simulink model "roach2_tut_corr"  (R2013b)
settings: Solver=VariableStepDiscrete  SolverMode=SingleTasking  StartTime=0.0  StopTime=100  RelTol=1e-3
undefined symbols (not defined in the file): add_latency, addr_width, Bit, bitfield, BitWidth, bram_latency, burst_size, casper_library_scopes, conv_latency, data_width, DelayLen, fan_latency, FFTSize, FFTStage, getfield, increment, led, Location, Lower, mult_latency, mux_latency, n_bits, n_bits_data, n_inputs, n_streams, n_taps, neg_latency, negate_latency, nsamples, pfb_size, pulse_len, reset_period, ROACH, ROACH2, snapshot, sx475t, sync_period, sync_period_bits, Upper, UseCounter, Width
libraries: xbsIndex_r4 x24444, casper_library_misc x73, xbsReplacements_r4 x34, casper_library_delays x14, xps_library x7
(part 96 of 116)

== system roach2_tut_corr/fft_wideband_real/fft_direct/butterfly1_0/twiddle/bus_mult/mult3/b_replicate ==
  in : Inport
  bussify : Subsystem  AncestorBlock=casper_library_flow_control/bus_create
  din0_0 : xbsIndex_r4/Delay  rst=off  infoeditControl=Selection of Reset will increase slice count due to use of real FFs and instead of SRLs  en=off  latency=1  dbl_ovrd=off  reg_retiming=off  block_type=delay
  din0_1 : xbsIndex_r4/Delay  rst=off  infoeditControl=Selection of Reset will increase slice count due to use of real FFs and instead of SRLs  en=off  latency=1  dbl_ovrd=off  reg_retiming=off  block_type=delay
  out : Outport
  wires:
  in/1 -> din0_0/1, din0_1/1
  din0_0/1 -> bussify/1(in1)
  din0_1/1 -> bussify/2(in2)
  bussify/1(bus_out) -> out/1

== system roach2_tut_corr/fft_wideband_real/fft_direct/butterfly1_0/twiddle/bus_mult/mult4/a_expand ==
  bus_in : Inport
  reinterpret{1..4} (4 alike) : xbsIndex_r4/Reinterpret  force_arith_type=on  arith_type="Signed  (2's comp)"  force_bin_pt=on  bin_pt=17  block_type=reinterpret
  slice1 : xbsIndex_r4/Slice  nbits=18  boolean_output=off  mode=Upper Bit Location + Width  bit1=-54  base1=MSB of Input  bit0=0  base0=LSB of Input  dbl_ovrd=off  block_type=slice
  slice2 : xbsIndex_r4/Slice  nbits=18  boolean_output=off  mode=Upper Bit Location + Width  bit1=-36  base1=MSB of Input  bit0=0  base0=LSB of Input  dbl_ovrd=off  block_type=slice
  slice3 : xbsIndex_r4/Slice  nbits=18  boolean_output=off  mode=Upper Bit Location + Width  bit1=-18  base1=MSB of Input  bit0=0  base0=LSB of Input  dbl_ovrd=off  block_type=slice
  slice4 : xbsIndex_r4/Slice  nbits=18  boolean_output=off  mode=Upper Bit Location + Width  bit1=0  base1=MSB of Input  bit0=0  base0=LSB of Input  dbl_ovrd=off  block_type=slice
  msb_out4 : Outport
  out3 : Outport  Port=2
  out2 : Outport  Port=3
  lsb_out1 : Outport  Port=4
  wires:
  bus_in/1 -> slice4/1, slice3/1, slice2/1, slice1/1
  slice4/1 -> reinterpret4/1
  reinterpret4/1 -> msb_out4/1
  slice3/1 -> reinterpret3/1
  reinterpret3/1 -> out3/1
  slice2/1 -> reinterpret2/1
  reinterpret2/1 -> out2/1
  slice1/1 -> reinterpret1/1
  reinterpret1/1 -> lsb_out1/1

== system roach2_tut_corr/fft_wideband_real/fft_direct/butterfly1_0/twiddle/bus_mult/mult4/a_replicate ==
  in : Inport
  bussify : Subsystem  AncestorBlock=casper_library_flow_control/bus_create
  din0_0 : xbsIndex_r4/Delay  rst=off  infoeditControl=Selection of Reset will increase slice count due to use of real FFs and instead of SRLs  en=off  latency=1  dbl_ovrd=off  reg_retiming=off  block_type=delay
  din0_1 : xbsIndex_r4/Delay  rst=off  infoeditControl=Selection of Reset will increase slice count due to use of real FFs and instead of SRLs  en=off  latency=1  dbl_ovrd=off  reg_retiming=off  block_type=delay
  out : Outport
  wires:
  in/1 -> din0_0/1, din0_1/1
  din0_0/1 -> bussify/1(in1)
  din0_1/1 -> bussify/2(in2)
  bussify/1(bus_out) -> out/1

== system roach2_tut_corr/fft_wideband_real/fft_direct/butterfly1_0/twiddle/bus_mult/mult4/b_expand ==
  bus_in : Inport
  reinterpret{1..4} (4 alike) : xbsIndex_r4/Reinterpret  force_arith_type=on  arith_type="Signed  (2's comp)"  force_bin_pt=on  bin_pt=17  block_type=reinterpret
  slice1 : xbsIndex_r4/Slice  nbits=18  boolean_output=off  mode=Upper Bit Location + Width  bit1=-54  base1=MSB of Input  bit0=0  base0=LSB of Input  dbl_ovrd=off  block_type=slice
  slice2 : xbsIndex_r4/Slice  nbits=18  boolean_output=off  mode=Upper Bit Location + Width  bit1=-36  base1=MSB of Input  bit0=0  base0=LSB of Input  dbl_ovrd=off  block_type=slice
  slice3 : xbsIndex_r4/Slice  nbits=18  boolean_output=off  mode=Upper Bit Location + Width  bit1=-18  base1=MSB of Input  bit0=0  base0=LSB of Input  dbl_ovrd=off  block_type=slice
  slice4 : xbsIndex_r4/Slice  nbits=18  boolean_output=off  mode=Upper Bit Location + Width  bit1=0  base1=MSB of Input  bit0=0  base0=LSB of Input  dbl_ovrd=off  block_type=slice
  msb_out4 : Outport
  out3 : Outport  Port=2
  out2 : Outport  Port=3
  lsb_out1 : Outport  Port=4
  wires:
  bus_in/1 -> slice4/1, slice3/1, slice2/1, slice1/1
  slice4/1 -> reinterpret4/1
  reinterpret4/1 -> msb_out4/1
  slice3/1 -> reinterpret3/1
  reinterpret3/1 -> out3/1
  slice2/1 -> reinterpret2/1
  reinterpret2/1 -> out2/1
  slice1/1 -> reinterpret1/1
  reinterpret1/1 -> lsb_out1/1

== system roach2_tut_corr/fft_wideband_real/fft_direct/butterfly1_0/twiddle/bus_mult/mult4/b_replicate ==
  in : Inport
  bussify : Subsystem  AncestorBlock=casper_library_flow_control/bus_create
  din0_0 : xbsIndex_r4/Delay  rst=off  infoeditControl=Selection of Reset will increase slice count due to use of real FFs and instead of SRLs  en=off  latency=1  dbl_ovrd=off  reg_retiming=off  block_type=delay
  din0_1 : xbsIndex_r4/Delay  rst=off  infoeditControl=Selection of Reset will increase slice count due to use of real FFs and instead of SRLs  en=off  latency=1  dbl_ovrd=off  reg_retiming=off  block_type=delay
  out : Outport
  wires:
  in/1 -> din0_0/1, din0_1/1
  din0_0/1 -> bussify/1(in1)
  din0_1/1 -> bussify/2(in2)
  bussify/1(bus_out) -> out/1

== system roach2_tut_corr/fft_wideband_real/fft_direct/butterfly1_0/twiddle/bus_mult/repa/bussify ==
  in1 : Inport
  reinterpret1 : xbsIndex_r4/Reinterpret  force_arith_type=on  arith_type=Unsigned  force_bin_pt=on  bin_pt=0  block_type=reinterpret
  bus_out : Outport
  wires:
  in1/1 -> reinterpret1/1
  reinterpret1/1 -> bus_out/1

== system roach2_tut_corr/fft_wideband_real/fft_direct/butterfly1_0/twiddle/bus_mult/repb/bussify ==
  in1 : Inport
  reinterpret1 : xbsIndex_r4/Reinterpret  force_arith_type=on  arith_type=Unsigned  force_bin_pt=on  bin_pt=0  block_type=reinterpret
  bus_out : Outport
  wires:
  in1/1 -> reinterpret1/1
  reinterpret1/1 -> bus_out/1

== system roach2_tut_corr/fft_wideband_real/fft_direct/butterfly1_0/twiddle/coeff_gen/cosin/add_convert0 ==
  theta : Inport
  misci : Inport  Port=2
  AddSub : xbsIndex_r4/AddSub  mode=Subtraction  use_carryin=off  use_carryout=off  en=off  latency=add_latency  precision=User Defined  arith_type=Unsigned  n_bits=10  bin_pt=0  quantization=Truncate  overflow=Wrap  dbl_ovrd=off  use_behavioral_HDL=off  hw_selection=Fabric  pipelined=on  block_type=addsub
  AddSub1 : xbsIndex_r4/AddSub  mode=Addition  use_carryin=off  use_carryout=off  en=off  latency=0  precision=User Defined  arith_type=Unsigned  n_bits=2  bin_pt=0  quantization=Truncate  overflow=Wrap  dbl_ovrd=off  use_behavioral_HDL=off  hw_selection=Fabric  pipelined=on  block_type=addsub
  AddSub5 : xbsIndex_r4/AddSub  mode=Addition  use_carryin=off  use_carryout=off  en=off  latency=0  precision=User Defined  arith_type=Unsigned  n_bits=2  bin_pt=0  quantization=Truncate  overflow=Wrap  dbl_ovrd=off  use_behavioral_HDL=off  hw_selection=Fabric  pipelined=off  block_type=addsub
  Concat : xbsIndex_r4/Concat  num_inputs=2  dbl_ovrd=off  block_type=concat
  Constant4 : xbsIndex_r4/Constant  const=512  gui_display_data_type=Fixed-point  arith_type=Unsigned  n_bits=10  bin_pt=0  preci_type=Single  exp_width=8  frac_width=24  explicit_period=off  period=1  equ=P=C  opselect=C  inp2=PCIN>>17  opr=+  inp1=P  carry=CIN  dbl_ovrd=off  block_type=constant
  Convert2 : xbsIndex_r4/Convert  gui_display_data_type=Fixed-point  arith_type=Unsigned  n_bits=9  bin_pt=0  float_type=Single  exp_bits=8  fraction_bits=24  quantization=Truncate  overflow=Saturate  en=off  latency=conv_latency  dbl_ovrd=off  pipeline=on  block_type=convert
  Delay1 : xbsIndex_r4/Delay  rst=off  infoeditControl=Selection of Reset will increase slice count due to use of real FFs and instead of SRLs  en=off  latency=mux_latency+add_latency+conv_latency  dbl_ovrd=off  reg_retiming=on  block_type=delay
  Delay13 : xbsIndex_r4/Delay  rst=off  infoeditControl=Selection of Reset will increase slice count due to use of real FFs and instead of SRLs  en=off  latency=add_latency  dbl_ovrd=off  reg_retiming=off  block_type=delay
  Delay14 : xbsIndex_r4/Delay  rst=off  infoeditControl=Selection of Reset will increase slice count due to use of real FFs and instead of SRLs  en=off  latency=add_latency  dbl_ovrd=off  reg_retiming=off  block_type=delay
  Delay2 : xbsIndex_r4/Delay  rst=off  infoeditControl=Selection of Reset will increase slice count due to use of real FFs and instead of SRLs  en=off  latency=add_latency+mux_latency+conv_latency  dbl_ovrd=off  reg_retiming=on  block_type=delay
  Mux : xbsIndex_r4/Mux  inputs=2  en=off  latency=mux_latency  precision=Full  arith_type=Unsigned  n_bits=16  bin_pt=14  quantization=Truncate  overflow=Wrap  dbl_ovrd=off  block_type=mux
  backwards : xbsIndex_r4/Slice  nbits=1  boolean_output=on  mode=Lower Bit Location + Width  bit1=0  base1=MSB of Input  bit0=0  base0=LSB of Input  dbl_ovrd=off  block_type=slice
  direction_offset : xbsIndex_r4/Constant  const=0  gui_display_data_type=Fixed-point  arith_type=Unsigned  n_bits=2  bin_pt=0  preci_type=Single  exp_width=8  frac_width=24  explicit_period=off  period=1  equ=P=C  opselect=C  inp2=PCIN>>17  opr=+  inp1=P  carry=CIN  dbl_ovrd=off  block_type=constant
  fluff : xbsIndex_r4/Concat  num_inputs=2  dbl_ovrd=off  block_type=concat
  invert : xbsIndex_r4/Slice  nbits=1  boolean_output=on  mode=Upper Bit Location + Width  bit1=0  base1=MSB of Input  bit0=0  base0=LSB of Input  dbl_ovrd=off  block_type=slice
  lookup : xbsIndex_r4/Slice  nbits=9  boolean_output=off  mode=Lower Bit Location + Width  bit1=0  base1=MSB of Input  bit0=0  base0=LSB of Input  dbl_ovrd=off  block_type=slice
  negate_offset : xbsIndex_r4/Constant  const=1  gui_display_data_type=Fixed-point  arith_type=Unsigned  n_bits=2  bin_pt=0  preci_type=Single  exp_width=8  frac_width=24  explicit_period=off  period=1  equ=P=C  opselect=C  inp2=PCIN>>17  opr=+  inp1=P  carry=CIN  dbl_ovrd=off  block_type=constant
  new_add : xbsIndex_r4/Slice  nbits=9  boolean_output=off  mode=Lower Bit Location + Width  bit1=0  base1=MSB of Input  bit0=0  base0=LSB of Input  dbl_ovrd=off  block_type=slice
  pad : xbsIndex_r4/Constant  const=0  gui_display_data_type=Fixed-point  arith_type=Unsigned  n_bits=2  bin_pt=0  preci_type=Single  exp_width=8  frac_width=24  explicit_period=off  period=1  equ=P=C  opselect=C  inp2=PCIN>>17  opr=+  inp1=P  carry=CIN  dbl_ovrd=off  block_type=constant
  quadrant : xbsIndex_r4/Slice  nbits=2  boolean_output=off  mode=Upper Bit Location + Width  bit1=0  base1=MSB of Input  bit0=0  base0=LSB of Input  dbl_ovrd=off  block_type=slice
  negate : Outport
  add : Outport  Port=2
  misco : Outport  Port=3
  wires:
  theta/1 -> fluff/2
  pad/1 -> fluff/1
  fluff/1 -> quadrant/1, lookup/1
  direction_offset/1 -> AddSub5/1
  quadrant/1 -> AddSub5/2, AddSub1/2
  lookup/1 -> Concat/2
  AddSub5/1 -> Concat/1, backwards/1
  Concat/1 -> new_add/1
  new_add/1 -> Delay14/1, AddSub/2
  Convert2/1 -> add/1
  backwards/1 -> Delay13/1
  Constant4/1 -> AddSub/1
  Delay13/1 -> Mux/1
  Delay14/1 -> Mux/2
  AddSub/1 -> Mux/3
  Mux/1 -> Convert2/1
  negate_offset/1 -> AddSub1/1
  AddSub1/1 -> invert/1
  invert/1 -> Delay2/1
  Delay2/1 -> negate/1
  misci/1 -> Delay1/1
  Delay1/1 -> misco/1

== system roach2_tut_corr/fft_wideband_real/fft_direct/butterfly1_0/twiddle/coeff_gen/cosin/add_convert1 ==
  theta : Inport
  misci : Inport  Port=2
  AddSub : xbsIndex_r4/AddSub  mode=Subtraction  use_carryin=off  use_carryout=off  en=off  latency=add_latency  precision=User Defined  arith_type=Unsigned  n_bits=10  bin_pt=0  quantization=Truncate  overflow=Wrap  dbl_ovrd=off  use_behavioral_HDL=off  hw_selection=Fabric  pipelined=on  block_type=addsub
  AddSub5 : xbsIndex_r4/AddSub  mode=Addition  use_carryin=off  use_carryout=off  en=off  latency=0  precision=User Defined  arith_type=Unsigned  n_bits=2  bin_pt=0  quantization=Truncate  overflow=Wrap  dbl_ovrd=off  use_behavioral_HDL=off  hw_selection=Fabric  pipelined=off  block_type=addsub
  Concat : xbsIndex_r4/Concat  num_inputs=2  dbl_ovrd=off  block_type=concat
  Constant4 : xbsIndex_r4/Constant  const=512  gui_display_data_type=Fixed-point  arith_type=Unsigned  n_bits=10  bin_pt=0  preci_type=Single  exp_width=8  frac_width=24  explicit_period=off  period=1  equ=P=C  opselect=C  inp2=PCIN>>17  opr=+  inp1=P  carry=CIN  dbl_ovrd=off  block_type=constant
  Convert2 : xbsIndex_r4/Convert  gui_display_data_type=Fixed-point  arith_type=Unsigned  n_bits=9  bin_pt=0  float_type=Single  exp_bits=8  fraction_bits=24  quantization=Truncate  overflow=Saturate  en=off  latency=conv_latency  dbl_ovrd=off  pipeline=on  block_type=convert
  Delay1 : xbsIndex_r4/Delay  rst=off  infoeditControl=Selection of Reset will increase slice count due to use of real FFs and instead of SRLs  en=off  latency=mux_latency+add_latency+conv_latency  dbl_ovrd=off  reg_retiming=on  block_type=delay
  Delay13 : xbsIndex_r4/Delay  rst=off  infoeditControl=Selection of Reset will increase slice count due to use of real FFs and instead of SRLs  en=off  latency=add_latency  dbl_ovrd=off  reg_retiming=off  block_type=delay
  Delay14 : xbsIndex_r4/Delay  rst=off  infoeditControl=Selection of Reset will increase slice count due to use of real FFs and instead of SRLs  en=off  latency=add_latency  dbl_ovrd=off  reg_retiming=off  block_type=delay
  Delay2 : xbsIndex_r4/Delay  rst=off  infoeditControl=Selection of Reset will increase slice count due to use of real FFs and instead of SRLs  en=off  latency=add_latency+mux_latency+conv_latency  dbl_ovrd=off  reg_retiming=on  block_type=delay
  Mux : xbsIndex_r4/Mux  inputs=2  en=off  latency=mux_latency  precision=Full  arith_type=Unsigned  n_bits=16  bin_pt=14  quantization=Truncate  overflow=Wrap  dbl_ovrd=off  block_type=mux
  backwards : xbsIndex_r4/Slice  nbits=1  boolean_output=on  mode=Lower Bit Location + Width  bit1=0  base1=MSB of Input  bit0=0  base0=LSB of Input  dbl_ovrd=off  block_type=slice
  direction_offset : xbsIndex_r4/Constant  const=0  gui_display_data_type=Fixed-point  arith_type=Unsigned  n_bits=2  bin_pt=0  preci_type=Single  exp_width=8  frac_width=24  explicit_period=off  period=1  equ=P=C  opselect=C  inp2=PCIN>>17  opr=+  inp1=P  carry=CIN  dbl_ovrd=off  block_type=constant
  fluff : xbsIndex_r4/Concat  num_inputs=2  dbl_ovrd=off  block_type=concat
  invert : xbsIndex_r4/Slice  nbits=1  boolean_output=on  mode=Upper Bit Location + Width  bit1=0  base1=MSB of Input  bit0=0  base0=LSB of Input  dbl_ovrd=off  block_type=slice
  lookup : xbsIndex_r4/Slice  nbits=9  boolean_output=off  mode=Lower Bit Location + Width  bit1=0  base1=MSB of Input  bit0=0  base0=LSB of Input  dbl_ovrd=off  block_type=slice
  new_add : xbsIndex_r4/Slice  nbits=9  boolean_output=off  mode=Lower Bit Location + Width  bit1=0  base1=MSB of Input  bit0=0  base0=LSB of Input  dbl_ovrd=off  block_type=slice
  pad : xbsIndex_r4/Constant  const=0  gui_display_data_type=Fixed-point  arith_type=Unsigned  n_bits=2  bin_pt=0  preci_type=Single  exp_width=8  frac_width=24  explicit_period=off  period=1  equ=P=C  opselect=C  inp2=PCIN>>17  opr=+  inp1=P  carry=CIN  dbl_ovrd=off  block_type=constant
  quadrant : xbsIndex_r4/Slice  nbits=2  boolean_output=off  mode=Upper Bit Location + Width  bit1=0  base1=MSB of Input  bit0=0  base0=LSB of Input  dbl_ovrd=off  block_type=slice
  negate : Outport
  add : Outport  Port=2
  misco : Outport  Port=3
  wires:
  theta/1 -> fluff/2
  pad/1 -> fluff/1
  fluff/1 -> quadrant/1, lookup/1
  direction_offset/1 -> AddSub5/1
  quadrant/1 -> AddSub5/2
  lookup/1 -> Concat/2
  AddSub5/1 -> Concat/1, backwards/1, invert/1
  Concat/1 -> new_add/1
  new_add/1 -> Delay14/1, AddSub/2
  Convert2/1 -> add/1
  backwards/1 -> Delay13/1
  Constant4/1 -> AddSub/1
  Delay13/1 -> Mux/1
  Delay14/1 -> Mux/2
  AddSub/1 -> Mux/3
  Mux/1 -> Convert2/1
  invert/1 -> Delay2/1
  Delay2/1 -> negate/1
  misci/1 -> Delay1/1
  Delay1/1 -> misco/1

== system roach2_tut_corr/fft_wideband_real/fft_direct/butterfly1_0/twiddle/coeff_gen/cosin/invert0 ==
  negate : Inport
  in : Inport  Port=2
  misci : Inport  Port=3
  Delay1 : xbsIndex_r4/Delay  rst=off  infoeditControl=Selection of Reset will increase slice count due to use of real FFs and instead of SRLs  en=off  latency=mux_latency+neg_latency  dbl_ovrd=off  reg_retiming=on  block_type=delay
  Delay20 : xbsIndex_r4/Delay  rst=off  infoeditControl=Selection of Reset will increase slice count due to use of real FFs and instead of SRLs  en=off  latency=neg_latency  dbl_ovrd=off  reg_retiming=on  block_type=delay
  Delay21 : xbsIndex_r4/Delay  rst=off  infoeditControl=Selection of Reset will increase slice count due to use of real FFs and instead of SRLs  en=off  latency=neg_latency  dbl_ovrd=off  reg_retiming=on  block_type=delay
  Negate : xbsIndex_r4/Negate  precision=User Defined  arith_type="Signed  (2's comp)"  n_bits=n_bits  bin_pt=bin_pt  quantization=Truncate  overflow=Saturate  en=off  latency=neg_latency  dbl_ovrd=off  block_type=negate
  mux : xbsIndex_r4/Mux  inputs=2  en=off  latency=mux_latency  precision=Full  arith_type=Unsigned  n_bits=16  bin_pt=14  quantization=Truncate  overflow=Wrap  dbl_ovrd=off  block_type=mux
  out : Outport
  misco : Outport  Port=2
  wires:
  misci/1 -> Delay1/1
  negate/1 -> Delay21/1
  in/1 -> Negate/1, Delay20/1
  Delay21/1 -> mux/1
  Delay20/1 -> mux/2
  Negate/1 -> mux/3
  mux/1 -> out/1
  Delay1/1 -> misco/1

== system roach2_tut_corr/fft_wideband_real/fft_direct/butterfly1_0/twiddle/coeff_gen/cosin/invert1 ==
  negate : Inport
  in : Inport  Port=2
  misci : Inport  Port=3
  Delay1 : xbsIndex_r4/Delay  rst=off  infoeditControl=Selection of Reset will increase slice count due to use of real FFs and instead of SRLs  en=off  latency=mux_latency+neg_latency  dbl_ovrd=off  reg_retiming=on  block_type=delay
  Delay20 : xbsIndex_r4/Delay  rst=off  infoeditControl=Selection of Reset will increase slice count due to use of real FFs and instead of SRLs  en=off  latency=neg_latency  dbl_ovrd=off  reg_retiming=on  block_type=delay
  Delay21 : xbsIndex_r4/Delay  rst=off  infoeditControl=Selection of Reset will increase slice count due to use of real FFs and instead of SRLs  en=off  latency=neg_latency  dbl_ovrd=off  reg_retiming=on  block_type=delay
  Negate : xbsIndex_r4/Negate  precision=User Defined  arith_type="Signed  (2's comp)"  n_bits=n_bits  bin_pt=bin_pt  quantization=Truncate  overflow=Saturate  en=off  latency=neg_latency  dbl_ovrd=off  block_type=negate
  mux : xbsIndex_r4/Mux  inputs=2  en=off  latency=mux_latency  precision=Full  arith_type=Unsigned  n_bits=16  bin_pt=14  quantization=Truncate  overflow=Wrap  dbl_ovrd=off  block_type=mux
  out : Outport
  misco : Outport  Port=2
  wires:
  misci/1 -> Delay1/1
  negate/1 -> Delay21/1
  in/1 -> Negate/1, Delay20/1
  Delay21/1 -> mux/1
  Delay20/1 -> mux/2
  Negate/1 -> mux/3
  mux/1 -> out/1
  Delay1/1 -> misco/1

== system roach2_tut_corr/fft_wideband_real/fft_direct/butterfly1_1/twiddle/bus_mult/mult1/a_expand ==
  bus_in : Inport
  reinterpret{1..4} (4 alike) : xbsIndex_r4/Reinterpret  force_arith_type=on  arith_type="Signed  (2's comp)"  force_bin_pt=on  bin_pt=17  block_type=reinterpret
  slice1 : xbsIndex_r4/Slice  nbits=18  boolean_output=off  mode=Upper Bit Location + Width  bit1=-54  base1=MSB of Input  bit0=0  base0=LSB of Input  dbl_ovrd=off  block_type=slice
  slice2 : xbsIndex_r4/Slice  nbits=18  boolean_output=off  mode=Upper Bit Location + Width  bit1=-36  base1=MSB of Input  bit0=0  base0=LSB of Input  dbl_ovrd=off  block_type=slice
  slice3 : xbsIndex_r4/Slice  nbits=18  boolean_output=off  mode=Upper Bit Location + Width  bit1=-18  base1=MSB of Input  bit0=0  base0=LSB of Input  dbl_ovrd=off  block_type=slice
  slice4 : xbsIndex_r4/Slice  nbits=18  boolean_output=off  mode=Upper Bit Location + Width  bit1=0  base1=MSB of Input  bit0=0  base0=LSB of Input  dbl_ovrd=off  block_type=slice
  msb_out4 : Outport
  out3 : Outport  Port=2
  out2 : Outport  Port=3
  lsb_out1 : Outport  Port=4
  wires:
  bus_in/1 -> slice4/1, slice3/1, slice2/1, slice1/1
  slice4/1 -> reinterpret4/1
  reinterpret4/1 -> msb_out4/1
  slice3/1 -> reinterpret3/1
  reinterpret3/1 -> out3/1
  slice2/1 -> reinterpret2/1
  reinterpret2/1 -> out2/1
  slice1/1 -> reinterpret1/1
  reinterpret1/1 -> lsb_out1/1

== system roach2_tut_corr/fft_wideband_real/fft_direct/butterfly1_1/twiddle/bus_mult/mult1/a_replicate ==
  in : Inport
  bussify : Subsystem  AncestorBlock=casper_library_flow_control/bus_create
  din0_0 : xbsIndex_r4/Delay  rst=off  infoeditControl=Selection of Reset will increase slice count due to use of real FFs and instead of SRLs  en=off  latency=1  dbl_ovrd=off  reg_retiming=off  block_type=delay
  din0_1 : xbsIndex_r4/Delay  rst=off  infoeditControl=Selection of Reset will increase slice count due to use of real FFs and instead of SRLs  en=off  latency=1  dbl_ovrd=off  reg_retiming=off  block_type=delay
  out : Outport
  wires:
  in/1 -> din0_0/1, din0_1/1
  din0_0/1 -> bussify/1(in1)
  din0_1/1 -> bussify/2(in2)
  bussify/1(bus_out) -> out/1

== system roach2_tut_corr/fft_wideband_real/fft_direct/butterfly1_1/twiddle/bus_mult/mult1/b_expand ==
  bus_in : Inport
  reinterpret{1..4} (4 alike) : xbsIndex_r4/Reinterpret  force_arith_type=on  arith_type="Signed  (2's comp)"  force_bin_pt=on  bin_pt=17  block_type=reinterpret
  slice1 : xbsIndex_r4/Slice  nbits=18  boolean_output=off  mode=Upper Bit Location + Width  bit1=-54  base1=MSB of Input  bit0=0  base0=LSB of Input  dbl_ovrd=off  block_type=slice
  slice2 : xbsIndex_r4/Slice  nbits=18  boolean_output=off  mode=Upper Bit Location + Width  bit1=-36  base1=MSB of Input  bit0=0  base0=LSB of Input  dbl_ovrd=off  block_type=slice
  slice3 : xbsIndex_r4/Slice  nbits=18  boolean_output=off  mode=Upper Bit Location + Width  bit1=-18  base1=MSB of Input  bit0=0  base0=LSB of Input  dbl_ovrd=off  block_type=slice
  slice4 : xbsIndex_r4/Slice  nbits=18  boolean_output=off  mode=Upper Bit Location + Width  bit1=0  base1=MSB of Input  bit0=0  base0=LSB of Input  dbl_ovrd=off  block_type=slice
  msb_out4 : Outport
  out3 : Outport  Port=2
  out2 : Outport  Port=3
  lsb_out1 : Outport  Port=4
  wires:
  bus_in/1 -> slice4/1, slice3/1, slice2/1, slice1/1
  slice4/1 -> reinterpret4/1
  reinterpret4/1 -> msb_out4/1
  slice3/1 -> reinterpret3/1
  reinterpret3/1 -> out3/1
  slice2/1 -> reinterpret2/1
  reinterpret2/1 -> out2/1
  slice1/1 -> reinterpret1/1
  reinterpret1/1 -> lsb_out1/1

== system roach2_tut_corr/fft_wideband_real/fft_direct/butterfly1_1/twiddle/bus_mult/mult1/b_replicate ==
  in : Inport
  bussify : Subsystem  AncestorBlock=casper_library_flow_control/bus_create
  din0_0 : xbsIndex_r4/Delay  rst=off  infoeditControl=Selection of Reset will increase slice count due to use of real FFs and instead of SRLs  en=off  latency=1  dbl_ovrd=off  reg_retiming=off  block_type=delay
  din0_1 : xbsIndex_r4/Delay  rst=off  infoeditControl=Selection of Reset will increase slice count due to use of real FFs and instead of SRLs  en=off  latency=1  dbl_ovrd=off  reg_retiming=off  block_type=delay
  out : Outport
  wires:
  in/1 -> din0_0/1, din0_1/1
  din0_0/1 -> bussify/1(in1)
  din0_1/1 -> bussify/2(in2)
  bussify/1(bus_out) -> out/1

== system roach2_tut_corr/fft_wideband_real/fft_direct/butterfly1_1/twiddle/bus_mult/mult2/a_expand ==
  bus_in : Inport
  reinterpret{1..4} (4 alike) : xbsIndex_r4/Reinterpret  force_arith_type=on  arith_type="Signed  (2's comp)"  force_bin_pt=on  bin_pt=17  block_type=reinterpret
  slice1 : xbsIndex_r4/Slice  nbits=18  boolean_output=off  mode=Upper Bit Location + Width  bit1=-54  base1=MSB of Input  bit0=0  base0=LSB of Input  dbl_ovrd=off  block_type=slice
  slice2 : xbsIndex_r4/Slice  nbits=18  boolean_output=off  mode=Upper Bit Location + Width  bit1=-36  base1=MSB of Input  bit0=0  base0=LSB of Input  dbl_ovrd=off  block_type=slice
  slice3 : xbsIndex_r4/Slice  nbits=18  boolean_output=off  mode=Upper Bit Location + Width  bit1=-18  base1=MSB of Input  bit0=0  base0=LSB of Input  dbl_ovrd=off  block_type=slice
  slice4 : xbsIndex_r4/Slice  nbits=18  boolean_output=off  mode=Upper Bit Location + Width  bit1=0  base1=MSB of Input  bit0=0  base0=LSB of Input  dbl_ovrd=off  block_type=slice
  msb_out4 : Outport
  out3 : Outport  Port=2
  out2 : Outport  Port=3
  lsb_out1 : Outport  Port=4
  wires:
  bus_in/1 -> slice4/1, slice3/1, slice2/1, slice1/1
  slice4/1 -> reinterpret4/1
  reinterpret4/1 -> msb_out4/1
  slice3/1 -> reinterpret3/1
  reinterpret3/1 -> out3/1
  slice2/1 -> reinterpret2/1
  reinterpret2/1 -> out2/1
  slice1/1 -> reinterpret1/1
  reinterpret1/1 -> lsb_out1/1

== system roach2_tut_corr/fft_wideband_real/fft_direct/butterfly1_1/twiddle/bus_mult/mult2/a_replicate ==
  in : Inport
  bussify : Subsystem  AncestorBlock=casper_library_flow_control/bus_create
  din0_0 : xbsIndex_r4/Delay  rst=off  infoeditControl=Selection of Reset will increase slice count due to use of real FFs and instead of SRLs  en=off  latency=1  dbl_ovrd=off  reg_retiming=off  block_type=delay
  din0_1 : xbsIndex_r4/Delay  rst=off  infoeditControl=Selection of Reset will increase slice count due to use of real FFs and instead of SRLs  en=off  latency=1  dbl_ovrd=off  reg_retiming=off  block_type=delay
  out : Outport
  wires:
  in/1 -> din0_0/1, din0_1/1
  din0_0/1 -> bussify/1(in1)
  din0_1/1 -> bussify/2(in2)
  bussify/1(bus_out) -> out/1

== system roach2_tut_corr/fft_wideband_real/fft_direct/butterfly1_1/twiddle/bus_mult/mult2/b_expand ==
  bus_in : Inport
  reinterpret{1..4} (4 alike) : xbsIndex_r4/Reinterpret  force_arith_type=on  arith_type="Signed  (2's comp)"  force_bin_pt=on  bin_pt=17  block_type=reinterpret
  slice1 : xbsIndex_r4/Slice  nbits=18  boolean_output=off  mode=Upper Bit Location + Width  bit1=-54  base1=MSB of Input  bit0=0  base0=LSB of Input  dbl_ovrd=off  block_type=slice
  slice2 : xbsIndex_r4/Slice  nbits=18  boolean_output=off  mode=Upper Bit Location + Width  bit1=-36  base1=MSB of Input  bit0=0  base0=LSB of Input  dbl_ovrd=off  block_type=slice
  slice3 : xbsIndex_r4/Slice  nbits=18  boolean_output=off  mode=Upper Bit Location + Width  bit1=-18  base1=MSB of Input  bit0=0  base0=LSB of Input  dbl_ovrd=off  block_type=slice
  slice4 : xbsIndex_r4/Slice  nbits=18  boolean_output=off  mode=Upper Bit Location + Width  bit1=0  base1=MSB of Input  bit0=0  base0=LSB of Input  dbl_ovrd=off  block_type=slice
  msb_out4 : Outport
  out3 : Outport  Port=2
  out2 : Outport  Port=3
  lsb_out1 : Outport  Port=4
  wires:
  bus_in/1 -> slice4/1, slice3/1, slice2/1, slice1/1
  slice4/1 -> reinterpret4/1
  reinterpret4/1 -> msb_out4/1
  slice3/1 -> reinterpret3/1
  reinterpret3/1 -> out3/1
  slice2/1 -> reinterpret2/1
  reinterpret2/1 -> out2/1
  slice1/1 -> reinterpret1/1
  reinterpret1/1 -> lsb_out1/1

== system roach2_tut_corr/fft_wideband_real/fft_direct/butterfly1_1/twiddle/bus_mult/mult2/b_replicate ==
  in : Inport
  bussify : Subsystem  AncestorBlock=casper_library_flow_control/bus_create
  din0_0 : xbsIndex_r4/Delay  rst=off  infoeditControl=Selection of Reset will increase slice count due to use of real FFs and instead of SRLs  en=off  latency=1  dbl_ovrd=off  reg_retiming=off  block_type=delay
  din0_1 : xbsIndex_r4/Delay  rst=off  infoeditControl=Selection of Reset will increase slice count due to use of real FFs and instead of SRLs  en=off  latency=1  dbl_ovrd=off  reg_retiming=off  block_type=delay
  out : Outport
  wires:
  in/1 -> din0_0/1, din0_1/1
  din0_0/1 -> bussify/1(in1)
  din0_1/1 -> bussify/2(in2)
  bussify/1(bus_out) -> out/1

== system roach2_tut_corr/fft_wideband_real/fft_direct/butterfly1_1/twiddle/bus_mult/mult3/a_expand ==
  bus_in : Inport
  reinterpret{1..4} (4 alike) : xbsIndex_r4/Reinterpret  force_arith_type=on  arith_type="Signed  (2's comp)"  force_bin_pt=on  bin_pt=17  block_type=reinterpret
  slice1 : xbsIndex_r4/Slice  nbits=18  boolean_output=off  mode=Upper Bit Location + Width  bit1=-54  base1=MSB of Input  bit0=0  base0=LSB of Input  dbl_ovrd=off  block_type=slice
  slice2 : xbsIndex_r4/Slice  nbits=18  boolean_output=off  mode=Upper Bit Location + Width  bit1=-36  base1=MSB of Input  bit0=0  base0=LSB of Input  dbl_ovrd=off  block_type=slice
  slice3 : xbsIndex_r4/Slice  nbits=18  boolean_output=off  mode=Upper Bit Location + Width  bit1=-18  base1=MSB of Input  bit0=0  base0=LSB of Input  dbl_ovrd=off  block_type=slice
  slice4 : xbsIndex_r4/Slice  nbits=18  boolean_output=off  mode=Upper Bit Location + Width  bit1=0  base1=MSB of Input  bit0=0  base0=LSB of Input  dbl_ovrd=off  block_type=slice
  msb_out4 : Outport
  out3 : Outport  Port=2
  out2 : Outport  Port=3
  lsb_out1 : Outport  Port=4
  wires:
  bus_in/1 -> slice4/1, slice3/1, slice2/1, slice1/1
  slice4/1 -> reinterpret4/1
  reinterpret4/1 -> msb_out4/1
  slice3/1 -> reinterpret3/1
  reinterpret3/1 -> out3/1
  slice2/1 -> reinterpret2/1
  reinterpret2/1 -> out2/1
  slice1/1 -> reinterpret1/1
  reinterpret1/1 -> lsb_out1/1

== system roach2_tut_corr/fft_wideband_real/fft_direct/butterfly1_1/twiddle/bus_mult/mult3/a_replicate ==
  in : Inport
  bussify : Subsystem  AncestorBlock=casper_library_flow_control/bus_create
  din0_0 : xbsIndex_r4/Delay  rst=off  infoeditControl=Selection of Reset will increase slice count due to use of real FFs and instead of SRLs  en=off  latency=1  dbl_ovrd=off  reg_retiming=off  block_type=delay
  din0_1 : xbsIndex_r4/Delay  rst=off  infoeditControl=Selection of Reset will increase slice count due to use of real FFs and instead of SRLs  en=off  latency=1  dbl_ovrd=off  reg_retiming=off  block_type=delay
  out : Outport
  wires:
  in/1 -> din0_0/1, din0_1/1
  din0_0/1 -> bussify/1(in1)
  din0_1/1 -> bussify/2(in2)
  bussify/1(bus_out) -> out/1

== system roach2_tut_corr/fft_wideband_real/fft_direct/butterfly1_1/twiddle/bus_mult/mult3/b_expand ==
  bus_in : Inport
  reinterpret{1..4} (4 alike) : xbsIndex_r4/Reinterpret  force_arith_type=on  arith_type="Signed  (2's comp)"  force_bin_pt=on  bin_pt=17  block_type=reinterpret
  slice1 : xbsIndex_r4/Slice  nbits=18  boolean_output=off  mode=Upper Bit Location + Width  bit1=-54  base1=MSB of Input  bit0=0  base0=LSB of Input  dbl_ovrd=off  block_type=slice
  slice2 : xbsIndex_r4/Slice  nbits=18  boolean_output=off  mode=Upper Bit Location + Width  bit1=-36  base1=MSB of Input  bit0=0  base0=LSB of Input  dbl_ovrd=off  block_type=slice
  slice3 : xbsIndex_r4/Slice  nbits=18  boolean_output=off  mode=Upper Bit Location + Width  bit1=-18  base1=MSB of Input  bit0=0  base0=LSB of Input  dbl_ovrd=off  block_type=slice
  slice4 : xbsIndex_r4/Slice  nbits=18  boolean_output=off  mode=Upper Bit Location + Width  bit1=0  base1=MSB of Input  bit0=0  base0=LSB of Input  dbl_ovrd=off  block_type=slice
  msb_out4 : Outport
  out3 : Outport  Port=2
  out2 : Outport  Port=3
  lsb_out1 : Outport  Port=4
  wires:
  bus_in/1 -> slice4/1, slice3/1, slice2/1, slice1/1
  slice4/1 -> reinterpret4/1
  reinterpret4/1 -> msb_out4/1
  slice3/1 -> reinterpret3/1
  reinterpret3/1 -> out3/1
  slice2/1 -> reinterpret2/1
  reinterpret2/1 -> out2/1
  slice1/1 -> reinterpret1/1
  reinterpret1/1 -> lsb_out1/1

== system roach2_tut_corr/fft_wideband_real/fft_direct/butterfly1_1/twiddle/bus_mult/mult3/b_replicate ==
  in : Inport
  bussify : Subsystem  AncestorBlock=casper_library_flow_control/bus_create
  din0_0 : xbsIndex_r4/Delay  rst=off  infoeditControl=Selection of Reset will increase slice count due to use of real FFs and instead of SRLs  en=off  latency=1  dbl_ovrd=off  reg_retiming=off  block_type=delay
  din0_1 : xbsIndex_r4/Delay  rst=off  infoeditControl=Selection of Reset will increase slice count due to use of real FFs and instead of SRLs  en=off  latency=1  dbl_ovrd=off  reg_retiming=off  block_type=delay
  out : Outport
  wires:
  in/1 -> din0_0/1, din0_1/1
  din0_0/1 -> bussify/1(in1)
  din0_1/1 -> bussify/2(in2)
  bussify/1(bus_out) -> out/1

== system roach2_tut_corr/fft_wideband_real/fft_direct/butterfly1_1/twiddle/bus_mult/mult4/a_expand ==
  bus_in : Inport
  reinterpret{1..4} (4 alike) : xbsIndex_r4/Reinterpret  force_arith_type=on  arith_type="Signed  (2's comp)"  force_bin_pt=on  bin_pt=17  block_type=reinterpret
  slice1 : xbsIndex_r4/Slice  nbits=18  boolean_output=off  mode=Upper Bit Location + Width  bit1=-54  base1=MSB of Input  bit0=0  base0=LSB of Input  dbl_ovrd=off  block_type=slice
  slice2 : xbsIndex_r4/Slice  nbits=18  boolean_output=off  mode=Upper Bit Location + Width  bit1=-36  base1=MSB of Input  bit0=0  base0=LSB of Input  dbl_ovrd=off  block_type=slice
  slice3 : xbsIndex_r4/Slice  nbits=18  boolean_output=off  mode=Upper Bit Location + Width  bit1=-18  base1=MSB of Input  bit0=0  base0=LSB of Input  dbl_ovrd=off  block_type=slice
  slice4 : xbsIndex_r4/Slice  nbits=18  boolean_output=off  mode=Upper Bit Location + Width  bit1=0  base1=MSB of Input  bit0=0  base0=LSB of Input  dbl_ovrd=off  block_type=slice
  msb_out4 : Outport
  out3 : Outport  Port=2
  out2 : Outport  Port=3
  lsb_out1 : Outport  Port=4
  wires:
  bus_in/1 -> slice4/1, slice3/1, slice2/1, slice1/1
  slice4/1 -> reinterpret4/1
  reinterpret4/1 -> msb_out4/1
  slice3/1 -> reinterpret3/1
  reinterpret3/1 -> out3/1
  slice2/1 -> reinterpret2/1
  reinterpret2/1 -> out2/1
  slice1/1 -> reinterpret1/1
  reinterpret1/1 -> lsb_out1/1

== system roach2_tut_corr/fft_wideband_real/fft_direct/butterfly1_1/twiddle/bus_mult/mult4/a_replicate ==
  in : Inport
  bussify : Subsystem  AncestorBlock=casper_library_flow_control/bus_create
  din0_0 : xbsIndex_r4/Delay  rst=off  infoeditControl=Selection of Reset will increase slice count due to use of real FFs and instead of SRLs  en=off  latency=1  dbl_ovrd=off  reg_retiming=off  block_type=delay
  din0_1 : xbsIndex_r4/Delay  rst=off  infoeditControl=Selection of Reset will increase slice count due to use of real FFs and instead of SRLs  en=off  latency=1  dbl_ovrd=off  reg_retiming=off  block_type=delay
  out : Outport
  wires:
  in/1 -> din0_0/1, din0_1/1
  din0_0/1 -> bussify/1(in1)
  din0_1/1 -> bussify/2(in2)
  bussify/1(bus_out) -> out/1

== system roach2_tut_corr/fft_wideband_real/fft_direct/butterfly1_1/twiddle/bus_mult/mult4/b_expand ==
  bus_in : Inport
  reinterpret{1..4} (4 alike) : xbsIndex_r4/Reinterpret  force_arith_type=on  arith_type="Signed  (2's comp)"  force_bin_pt=on  bin_pt=17  block_type=reinterpret
  slice1 : xbsIndex_r4/Slice  nbits=18  boolean_output=off  mode=Upper Bit Location + Width  bit1=-54  base1=MSB of Input  bit0=0  base0=LSB of Input  dbl_ovrd=off  block_type=slice
  slice2 : xbsIndex_r4/Slice  nbits=18  boolean_output=off  mode=Upper Bit Location + Width  bit1=-36  base1=MSB of Input  bit0=0  base0=LSB of Input  dbl_ovrd=off  block_type=slice
  slice3 : xbsIndex_r4/Slice  nbits=18  boolean_output=off  mode=Upper Bit Location + Width  bit1=-18  base1=MSB of Input  bit0=0  base0=LSB of Input  dbl_ovrd=off  block_type=slice
  slice4 : xbsIndex_r4/Slice  nbits=18  boolean_output=off  mode=Upper Bit Location + Width  bit1=0  base1=MSB of Input  bit0=0  base0=LSB of Input  dbl_ovrd=off  block_type=slice
  msb_out4 : Outport
  out3 : Outport  Port=2
  out2 : Outport  Port=3
  lsb_out1 : Outport  Port=4
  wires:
  bus_in/1 -> slice4/1, slice3/1, slice2/1, slice1/1
  slice4/1 -> reinterpret4/1
  reinterpret4/1 -> msb_out4/1
  slice3/1 -> reinterpret3/1
  reinterpret3/1 -> out3/1
  slice2/1 -> reinterpret2/1
  reinterpret2/1 -> out2/1
  slice1/1 -> reinterpret1/1
  reinterpret1/1 -> lsb_out1/1

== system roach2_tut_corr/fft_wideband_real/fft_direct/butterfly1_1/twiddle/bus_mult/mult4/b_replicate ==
  in : Inport
  bussify : Subsystem  AncestorBlock=casper_library_flow_control/bus_create
  din0_0 : xbsIndex_r4/Delay  rst=off  infoeditControl=Selection of Reset will increase slice count due to use of real FFs and instead of SRLs  en=off  latency=1  dbl_ovrd=off  reg_retiming=off  block_type=delay
  din0_1 : xbsIndex_r4/Delay  rst=off  infoeditControl=Selection of Reset will increase slice count due to use of real FFs and instead of SRLs  en=off  latency=1  dbl_ovrd=off  reg_retiming=off  block_type=delay
  out : Outport
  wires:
  in/1 -> din0_0/1, din0_1/1
  din0_0/1 -> bussify/1(in1)
  din0_1/1 -> bussify/2(in2)
  bussify/1(bus_out) -> out/1

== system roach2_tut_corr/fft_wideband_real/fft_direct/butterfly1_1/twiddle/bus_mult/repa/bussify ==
  in1 : Inport
  reinterpret1 : xbsIndex_r4/Reinterpret  force_arith_type=on  arith_type=Unsigned  force_bin_pt=on  bin_pt=0  block_type=reinterpret
  bus_out : Outport
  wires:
  in1/1 -> reinterpret1/1
  reinterpret1/1 -> bus_out/1

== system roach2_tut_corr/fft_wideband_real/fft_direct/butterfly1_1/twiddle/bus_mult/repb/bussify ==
  in1 : Inport
  reinterpret1 : xbsIndex_r4/Reinterpret  force_arith_type=on  arith_type=Unsigned  force_bin_pt=on  bin_pt=0  block_type=reinterpret
  bus_out : Outport
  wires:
  in1/1 -> reinterpret1/1
  reinterpret1/1 -> bus_out/1

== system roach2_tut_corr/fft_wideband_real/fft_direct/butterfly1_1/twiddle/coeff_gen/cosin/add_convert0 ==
  theta : Inport
  misci : Inport  Port=2
  AddSub : xbsIndex_r4/AddSub  mode=Subtraction  use_carryin=off  use_carryout=off  en=off  latency=add_latency  precision=User Defined  arith_type=Unsigned  n_bits=10  bin_pt=0  quantization=Truncate  overflow=Wrap  dbl_ovrd=off  use_behavioral_HDL=off  hw_selection=Fabric  pipelined=on  block_type=addsub
  AddSub5 : xbsIndex_r4/AddSub  mode=Addition  use_carryin=off  use_carryout=off  en=off  latency=0  precision=User Defined  arith_type=Unsigned  n_bits=2  bin_pt=0  quantization=Truncate  overflow=Wrap  dbl_ovrd=off  use_behavioral_HDL=off  hw_selection=Fabric  pipelined=off  block_type=addsub
  Concat : xbsIndex_r4/Concat  num_inputs=2  dbl_ovrd=off  block_type=concat
  Constant4 : xbsIndex_r4/Constant  const=512  gui_display_data_type=Fixed-point  arith_type=Unsigned  n_bits=10  bin_pt=0  preci_type=Single  exp_width=8  frac_width=24  explicit_period=off  period=1  equ=P=C  opselect=C  inp2=PCIN>>17  opr=+  inp1=P  carry=CIN  dbl_ovrd=off  block_type=constant
  Convert2 : xbsIndex_r4/Convert  gui_display_data_type=Fixed-point  arith_type=Unsigned  n_bits=9  bin_pt=0  float_type=Single  exp_bits=8  fraction_bits=24  quantization=Truncate  overflow=Saturate  en=off  latency=conv_latency  dbl_ovrd=off  pipeline=on  block_type=convert
  Delay1 : xbsIndex_r4/Delay  rst=off  infoeditControl=Selection of Reset will increase slice count due to use of real FFs and instead of SRLs  en=off  latency=mux_latency+add_latency+conv_latency  dbl_ovrd=off  reg_retiming=on  block_type=delay
  Delay13 : xbsIndex_r4/Delay  rst=off  infoeditControl=Selection of Reset will increase slice count due to use of real FFs and instead of SRLs  en=off  latency=add_latency  dbl_ovrd=off  reg_retiming=off  block_type=delay
  Delay14 : xbsIndex_r4/Delay  rst=off  infoeditControl=Selection of Reset will increase slice count due to use of real FFs and instead of SRLs  en=off  latency=add_latency  dbl_ovrd=off  reg_retiming=off  block_type=delay
  Delay2 : xbsIndex_r4/Delay  rst=off  infoeditControl=Selection of Reset will increase slice count due to use of real FFs and instead of SRLs  en=off  latency=add_latency+mux_latency+conv_latency  dbl_ovrd=off  reg_retiming=on  block_type=delay
  Mux : xbsIndex_r4/Mux  inputs=2  en=off  latency=mux_latency  precision=Full  arith_type=Unsigned  n_bits=16  bin_pt=14  quantization=Truncate  overflow=Wrap  dbl_ovrd=off  block_type=mux
  backwards : xbsIndex_r4/Slice  nbits=1  boolean_output=on  mode=Lower Bit Location + Width  bit1=0  base1=MSB of Input  bit0=0  base0=LSB of Input  dbl_ovrd=off  block_type=slice
  direction_offset : xbsIndex_r4/Constant  const=0  gui_display_data_type=Fixed-point  arith_type=Unsigned  n_bits=2  bin_pt=0  preci_type=Single  exp_width=8  frac_width=24  explicit_period=off  period=1  equ=P=C  opselect=C  inp2=PCIN>>17  opr=+  inp1=P  carry=CIN  dbl_ovrd=off  block_type=constant
  fluff : xbsIndex_r4/Concat  num_inputs=2  dbl_ovrd=off  block_type=concat
  invert : xbsIndex_r4/Slice  nbits=1  boolean_output=on  mode=Upper Bit Location + Width  bit1=0  base1=MSB of Input  bit0=0  base0=LSB of Input  dbl_ovrd=off  block_type=slice
  lookup : xbsIndex_r4/Slice  nbits=9  boolean_output=off  mode=Lower Bit Location + Width  bit1=0  base1=MSB of Input  bit0=0  base0=LSB of Input  dbl_ovrd=off  block_type=slice
  new_add : xbsIndex_r4/Slice  nbits=9  boolean_output=off  mode=Lower Bit Location + Width  bit1=0  base1=MSB of Input  bit0=0  base0=LSB of Input  dbl_ovrd=off  block_type=slice
  pad : xbsIndex_r4/Constant  const=0  gui_display_data_type=Fixed-point  arith_type=Unsigned  n_bits=2  bin_pt=0  preci_type=Single  exp_width=8  frac_width=24  explicit_period=off  period=1  equ=P=C  opselect=C  inp2=PCIN>>17  opr=+  inp1=P  carry=CIN  dbl_ovrd=off  block_type=constant
  quadrant : xbsIndex_r4/Slice  nbits=2  boolean_output=off  mode=Upper Bit Location + Width  bit1=0  base1=MSB of Input  bit0=0  base0=LSB of Input  dbl_ovrd=off  block_type=slice
  negate : Outport
  add : Outport  Port=2
  misco : Outport  Port=3
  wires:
  theta/1 -> fluff/2
  pad/1 -> fluff/1
  fluff/1 -> quadrant/1, lookup/1
  direction_offset/1 -> AddSub5/1
  quadrant/1 -> AddSub5/2
  lookup/1 -> Concat/2
  AddSub5/1 -> Concat/1, backwards/1, invert/1
  Concat/1 -> new_add/1
  new_add/1 -> Delay14/1, AddSub/2
  Convert2/1 -> add/1
  backwards/1 -> Delay13/1
  Constant4/1 -> AddSub/1
  Delay13/1 -> Mux/1
  Delay14/1 -> Mux/2
  AddSub/1 -> Mux/3
  Mux/1 -> Convert2/1
  invert/1 -> Delay2/1
  Delay2/1 -> negate/1
  misci/1 -> Delay1/1
  Delay1/1 -> misco/1

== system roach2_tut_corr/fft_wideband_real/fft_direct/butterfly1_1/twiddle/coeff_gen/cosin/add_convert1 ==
  theta : Inport
  misci : Inport  Port=2
  AddSub : xbsIndex_r4/AddSub  mode=Subtraction  use_carryin=off  use_carryout=off  en=off  latency=add_latency  precision=User Defined  arith_type=Unsigned  n_bits=10  bin_pt=0  quantization=Truncate  overflow=Wrap  dbl_ovrd=off  use_behavioral_HDL=off  hw_selection=Fabric  pipelined=on  block_type=addsub
  AddSub1 : xbsIndex_r4/AddSub  mode=Addition  use_carryin=off  use_carryout=off  en=off  latency=0  precision=User Defined  arith_type=Unsigned  n_bits=2  bin_pt=0  quantization=Truncate  overflow=Wrap  dbl_ovrd=off  use_behavioral_HDL=off  hw_selection=Fabric  pipelined=on  block_type=addsub
  AddSub5 : xbsIndex_r4/AddSub  mode=Addition  use_carryin=off  use_carryout=off  en=off  latency=0  precision=User Defined  arith_type=Unsigned  n_bits=2  bin_pt=0  quantization=Truncate  overflow=Wrap  dbl_ovrd=off  use_behavioral_HDL=off  hw_selection=Fabric  pipelined=off  block_type=addsub
  Concat : xbsIndex_r4/Concat  num_inputs=2  dbl_ovrd=off  block_type=concat
  Constant4 : xbsIndex_r4/Constant  const=512  gui_display_data_type=Fixed-point  arith_type=Unsigned  n_bits=10  bin_pt=0  preci_type=Single  exp_width=8  frac_width=24  explicit_period=off  period=1  equ=P=C  opselect=C  inp2=PCIN>>17  opr=+  inp1=P  carry=CIN  dbl_ovrd=off  block_type=constant
  Convert2 : xbsIndex_r4/Convert  gui_display_data_type=Fixed-point  arith_type=Unsigned  n_bits=9  bin_pt=0  float_type=Single  exp_bits=8  fraction_bits=24  quantization=Truncate  overflow=Saturate  en=off  latency=conv_latency  dbl_ovrd=off  pipeline=on  block_type=convert
  Delay1 : xbsIndex_r4/Delay  rst=off  infoeditControl=Selection of Reset will increase slice count due to use of real FFs and instead of SRLs  en=off  latency=mux_latency+add_latency+conv_latency  dbl_ovrd=off  reg_retiming=on  block_type=delay
  Delay13 : xbsIndex_r4/Delay  rst=off  infoeditControl=Selection of Reset will increase slice count due to use of real FFs and instead of SRLs  en=off  latency=add_latency  dbl_ovrd=off  reg_retiming=off  block_type=delay
  Delay14 : xbsIndex_r4/Delay  rst=off  infoeditControl=Selection of Reset will increase slice count due to use of real FFs and instead of SRLs  en=off  latency=add_latency  dbl_ovrd=off  reg_retiming=off  block_type=delay
  Delay2 : xbsIndex_r4/Delay  rst=off  infoeditControl=Selection of Reset will increase slice count due to use of real FFs and instead of SRLs  en=off  latency=add_latency+mux_latency+conv_latency  dbl_ovrd=off  reg_retiming=on  block_type=delay
  Mux : xbsIndex_r4/Mux  inputs=2  en=off  latency=mux_latency  precision=Full  arith_type=Unsigned  n_bits=16  bin_pt=14  quantization=Truncate  overflow=Wrap  dbl_ovrd=off  block_type=mux
  backwards : xbsIndex_r4/Slice  nbits=1  boolean_output=on  mode=Lower Bit Location + Width  bit1=0  base1=MSB of Input  bit0=0  base0=LSB of Input  dbl_ovrd=off  block_type=slice
  direction_offset : xbsIndex_r4/Constant  const=0  gui_display_data_type=Fixed-point  arith_type=Unsigned  n_bits=2  bin_pt=0  preci_type=Single  exp_width=8  frac_width=24  explicit_period=off  period=1  equ=P=C  opselect=C  inp2=PCIN>>17  opr=+  inp1=P  carry=CIN  dbl_ovrd=off  block_type=constant
  fluff : xbsIndex_r4/Concat  num_inputs=2  dbl_ovrd=off  block_type=concat
  invert : xbsIndex_r4/Slice  nbits=1  boolean_output=on  mode=Upper Bit Location + Width  bit1=0  base1=MSB of Input  bit0=0  base0=LSB of Input  dbl_ovrd=off  block_type=slice
  lookup : xbsIndex_r4/Slice  nbits=9  boolean_output=off  mode=Lower Bit Location + Width  bit1=0  base1=MSB of Input  bit0=0  base0=LSB of Input  dbl_ovrd=off  block_type=slice
  negate_offset : xbsIndex_r4/Constant  const=1  gui_display_data_type=Fixed-point  arith_type=Unsigned  n_bits=2  bin_pt=0  preci_type=Single  exp_width=8  frac_width=24  explicit_period=off  period=1  equ=P=C  opselect=C  inp2=PCIN>>17  opr=+  inp1=P  carry=CIN  dbl_ovrd=off  block_type=constant
  new_add : xbsIndex_r4/Slice  nbits=9  boolean_output=off  mode=Lower Bit Location + Width  bit1=0  base1=MSB of Input  bit0=0  base0=LSB of Input  dbl_ovrd=off  block_type=slice
  pad : xbsIndex_r4/Constant  const=0  gui_display_data_type=Fixed-point  arith_type=Unsigned  n_bits=2  bin_pt=0  preci_type=Single  exp_width=8  frac_width=24  explicit_period=off  period=1  equ=P=C  opselect=C  inp2=PCIN>>17  opr=+  inp1=P  carry=CIN  dbl_ovrd=off  block_type=constant
  quadrant : xbsIndex_r4/Slice  nbits=2  boolean_output=off  mode=Upper Bit Location + Width  bit1=0  base1=MSB of Input  bit0=0  base0=LSB of Input  dbl_ovrd=off  block_type=slice
  negate : Outport
  add : Outport  Port=2
  misco : Outport  Port=3
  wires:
  theta/1 -> fluff/2
  pad/1 -> fluff/1
  fluff/1 -> quadrant/1, lookup/1
  direction_offset/1 -> AddSub5/1
  quadrant/1 -> AddSub5/2, AddSub1/2
  lookup/1 -> Concat/2
  AddSub5/1 -> Concat/1, backwards/1
  Concat/1 -> new_add/1
  new_add/1 -> Delay14/1, AddSub/2
  Convert2/1 -> add/1
  backwards/1 -> Delay13/1
  Constant4/1 -> AddSub/1
  Delay13/1 -> Mux/1
  Delay14/1 -> Mux/2
  AddSub/1 -> Mux/3
  Mux/1 -> Convert2/1
  negate_offset/1 -> AddSub1/1
  AddSub1/1 -> invert/1
  invert/1 -> Delay2/1
  Delay2/1 -> negate/1
  misci/1 -> Delay1/1
  Delay1/1 -> misco/1

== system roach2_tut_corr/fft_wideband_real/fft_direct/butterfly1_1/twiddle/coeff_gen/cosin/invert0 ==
  negate : Inport
  in : Inport  Port=2
  misci : Inport  Port=3
  Delay1 : xbsIndex_r4/Delay  rst=off  infoeditControl=Selection of Reset will increase slice count due to use of real FFs and instead of SRLs  en=off  latency=mux_latency+neg_latency  dbl_ovrd=off  reg_retiming=on  block_type=delay
  Delay20 : xbsIndex_r4/Delay  rst=off  infoeditControl=Selection of Reset will increase slice count due to use of real FFs and instead of SRLs  en=off  latency=neg_latency  dbl_ovrd=off  reg_retiming=on  block_type=delay
  Delay21 : xbsIndex_r4/Delay  rst=off  infoeditControl=Selection of Reset will increase slice count due to use of real FFs and instead of SRLs  en=off  latency=neg_latency  dbl_ovrd=off  reg_retiming=on  block_type=delay
  Negate : xbsIndex_r4/Negate  precision=User Defined  arith_type="Signed  (2's comp)"  n_bits=n_bits  bin_pt=bin_pt  quantization=Truncate  overflow=Saturate  en=off  latency=neg_latency  dbl_ovrd=off  block_type=negate
  mux : xbsIndex_r4/Mux  inputs=2  en=off  latency=mux_latency  precision=Full  arith_type=Unsigned  n_bits=16  bin_pt=14  quantization=Truncate  overflow=Wrap  dbl_ovrd=off  block_type=mux
  out : Outport
  misco : Outport  Port=2
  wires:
  misci/1 -> Delay1/1
  negate/1 -> Delay21/1
  in/1 -> Negate/1, Delay20/1
  Delay21/1 -> mux/1
  Delay20/1 -> mux/2
  Negate/1 -> mux/3
  mux/1 -> out/1
  Delay1/1 -> misco/1
